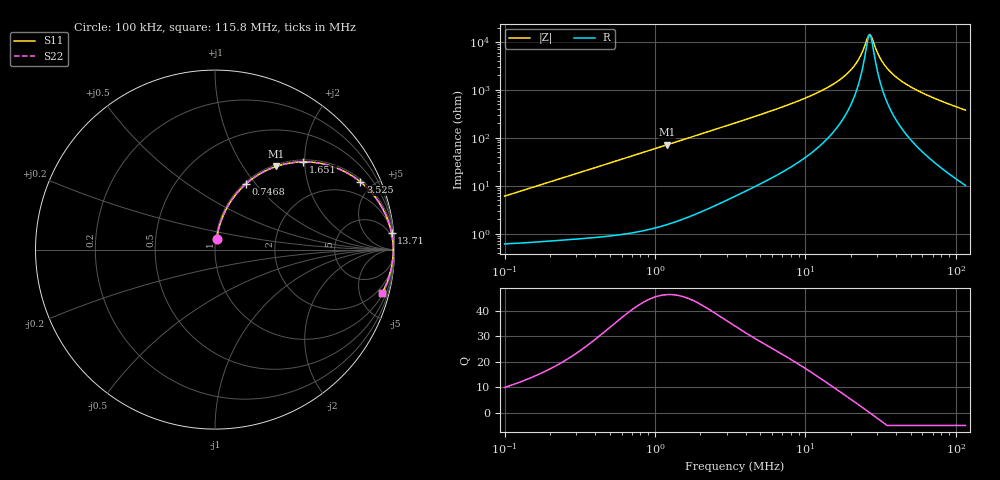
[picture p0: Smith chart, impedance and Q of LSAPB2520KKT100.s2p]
! LSAPB2520KKT100  S-PARAMETER MODEL  ( General Type )
! Model Generated by TAIYO YUDEN Corporation (http://www.ty-top.com)
! Version 1.0
! TAIYO YUDEN Control No. 171016NI43SB-FBB
! Copyright(c) 2017 TAIYO YUDEN CO.,LTD. All Rights Reserved.
! Product Description (link to TY-COMPAS)
! https://ds.yuden.co.jp/TYCOMPAS/or/detail?pn=LSAPB2520KKT100M&u=M
! Products Name : Inductors
! Characteristics :
!  Inductance : 10 uH , SRF(min) : -Hz , DC Resistance(max) : 0.65 Ohm
!  Rated Current : Saturation :1100 mA , Temp Rise : 750 mA (40 degC)
!  Case Size : 2.5 x 2.0 / 0.098 x 0.079 [mm/inch] , Thickness : 1 / 0.039 [mm/inch]
!  (Conditions: Temperature = 25 degC , DC Bias Current/Voltage = 0A / 0V)
! External Node Assignments :
!  1  o---GGG---o  2
! GND o---------o GND
! Frequency Range : 0.1MHz  -  115.823372MHz  [ 402 STEP ]
# MHz S RI R 50
! Freq[MHz].  S11 Real  S11 Imag  S21 Real  S21 Imag  S12 Real  S12 Imag  S22 Real  S22 Imag
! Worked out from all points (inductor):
!   401 points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, 100 kHz to 115.8 MHz, reference 50 ohm
!   read as one part in series: L = 9.58 uH near 103.6 kHz
!   highest Q = 46.2 at 1.202 MHz (marker M1), where L = 9.45 uH
!   self-resonance near 26.33 MHz
!   S11 on the Smith chart (normalised r, x): 100 kHz: 1.01, +0.12; 746.8 kHz: 1.02, +0.89; 1.651 MHz: 1.04, +1.96; 3.525 MHz: 1.13, +4.22; 13.71 MHz: 3, +21; 115.8 MHz: 1.20, -7.57
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0.1  0.00963 0.0594  0.9904 -0.0594  0.9904 -0.0594  0.00963 0.0594
0.325976  0.0434 0.1845  0.9566 -0.1845  0.9566 -0.1845  0.0434 0.1845
0.746761  0.1705 0.3642  0.8295 -0.3642  0.8295 -0.3642  0.1705 0.3642
1.062605  0.2891 0.4426  0.7109 -0.4426  0.7109 -0.4426  0.2891 0.4426
1.202232  0.3411 0.4634  0.6589 -0.4634  0.6589 -0.4634  0.3411 0.4634
1.651426  0.4908 0.4889  0.5092 -0.4889  0.5092 -0.4889  0.4908 0.4889
3.463838  0.8041 0.3823  0.1959 -0.3823  0.1959 -0.3823  0.8041 0.3823
3.52547  0.8095 0.378  0.1905 -0.378  0.1905 -0.378  0.8095 0.378
5.879526  0.9203 0.252  0.0797 -0.252  0.0797 -0.252  0.9203 0.252
11.09389  0.976 0.1243  0.024 -0.1243  0.024 -0.1243  0.976 0.1243
13.70875  0.984 0.0905  0.016 -0.0905  0.016 -0.0905  0.984 0.0905
17.24135  0.9893 0.0574  0.0107 -0.0574  0.0107 -0.0574  0.9893 0.0574
20.56677  0.9917 0.0338  0.00828 -0.0338  0.00828 -0.0338  0.9917 0.0338
22.86247  0.9926 0.0201  0.00744 -0.0201  0.00744 -0.0201  0.9926 0.0201
25.86661  0.993 0.00435  0.00697 -0.00435  0.00697 -0.00435  0.993 0.00435
26.79529  0.9931 -0.000138  0.00693 0.000138  0.00693 0.000138  0.9931 -0.000138
27.75732  0.9931 -0.00462  0.00694 0.00462  0.00694 0.00462  0.9931 -0.00462
31.96343  0.9926 -0.0227  0.00737 0.0227  0.00737 0.0227  0.9926 -0.0227
36.16345  0.9917 -0.0388  0.00833 0.0388  0.00833 0.0388  0.9917 -0.0388
43.13847  0.9892 -0.0628  0.0108 0.0628  0.0108 0.0628  0.9892 -0.0628
55.22015  0.9832 -0.0994  0.0168 0.0994  0.0168 0.0994  0.9832 -0.0994
115.8234  0.929 -0.2437  0.071 0.2437  0.071 0.2437  0.929 -0.2437
